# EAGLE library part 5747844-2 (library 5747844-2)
09 MSFL RCPT RA 318 (FM,BL) Source: Datasheet
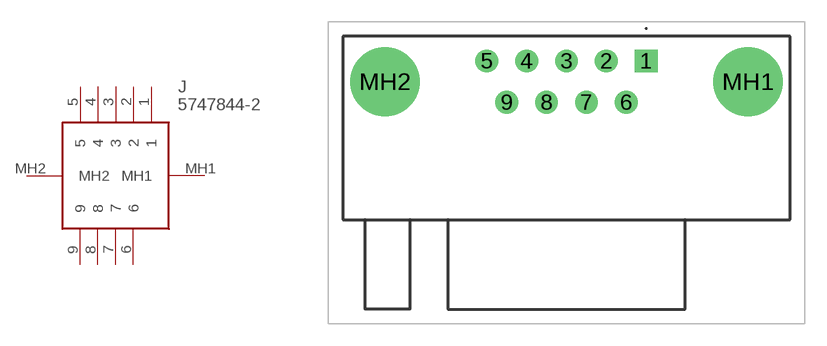
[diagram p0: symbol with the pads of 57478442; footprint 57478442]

Designator prefix J

## 5747844-2 (Arrow_Part_Number: 5747844-2; Arrow_Price-Stock: https://www.arrow.com/en/products/5747844-2/te-connectivity?region=nac; Description: 09 MSFL RCPT RA 318 (FM,BL); Height: 12.9286mm; Manufacturer_Name: TE Connectivity; Manufacturer_Part_Number: 5747844-2; Mouser_Part_Number: 571-5747844-2; Mouser_Price-Stock: https://www.mouser.co.uk/ProductDetail/TE-Connectivity/5747844-2?qs=DUjmvCJSYRCtNU6HMUj1IQ%3D%3D)  [57478442]
1  1
2  2
3  3
4  4
5  5
6  6
7  7
8  8
9  9
MH1  MH1
MH2  MH2

## Footprint 57478442 (pad centres in mm)
5747844-2-4
drill 1.041 pad 1.562 square: 1 0,0
drill 1.041 pad 1.562: 2 -2.743,0; 3 -5.486,0; 4 -8.23,0; 5 -10.973,0; 6 -1.372,-2.845; 7 -4.115,-2.845; 8 -6.858,-2.845; 9 -9.601,-2.845
drill 3.175 pad 4.762: MH1 7.01,-1.422; MH2 -17.983,-1.422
